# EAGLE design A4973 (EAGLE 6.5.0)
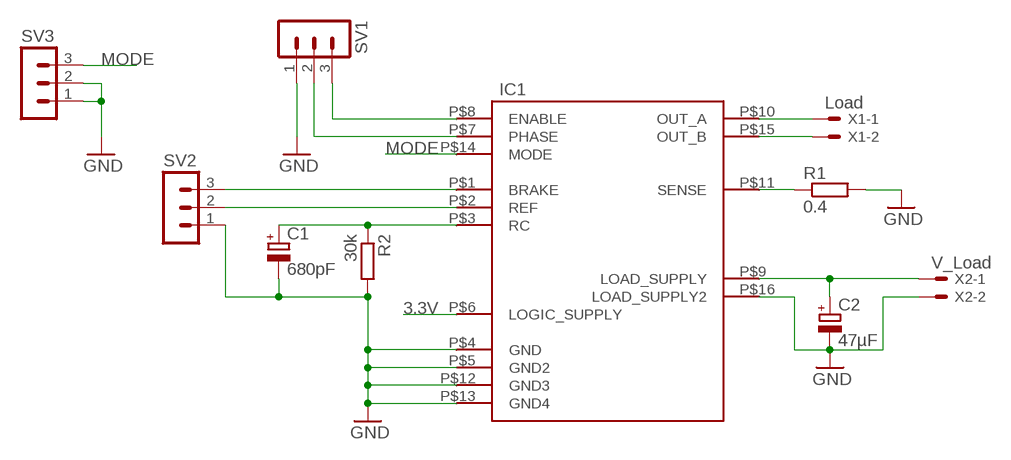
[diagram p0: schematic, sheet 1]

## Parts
C1  680pF  CPOL-EU153CLV-0405  [153CLV-0405]
C2  47µF  CPOL-EU153CLV-0405  [153CLV-0405]
IC1  A4973  [SOICW-16]
R1  0.4  R-EU_R1206  [R1206]
R2  30k  R-EU_R1206  [R1206]
SV1  MA03-1  [MA03-1]
SV2  MA03-1  [MA03-1]
SV3  MA03-1  [MA03-1]
X1  Load  22-23-2021  [22-23-2021]
X2  V_Load  22-23-2021  [22-23-2021]

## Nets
3.3V: IC1.P$6(LOGIC_SUPPLY)
GND: C1.- C2.- IC1.P$4(GND) IC1.P$5(GND2) IC1.P$12(GND3) IC1.P$13(GND4) IC1.P$16(LOAD_SUPPLY2) R1.2 R2.2 SV1.1 SV2.1 SV3.1 SV3.2 X2.2
MODE: IC1.P$14(MODE) SV3.3
N$1: IC1.P$8(ENABLE) SV1.3
N$2: IC1.P$7(PHASE) SV1.2
N$4: IC1.P$10(OUT_A) X1.1
N$5: IC1.P$15(OUT_B) X1.2
N$6: IC1.P$11(SENSE) R1.1
N$7: C1.+ IC1.P$3(RC) R2.1
N$8: C2.+ IC1.P$9(LOAD_SUPPLY) X2.1
N$9: IC1.P$1(BRAKE) SV2.3
N$10: IC1.P$2(REF) SV2.2

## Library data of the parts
C1 C2 = rcl:CPOL-EU: POLARIZED CAPACITOR, European symbol
IC1 = robust:A4973
R1 R2 = rcl:R-EU_: RESISTOR, European symbol
SV1-SV3 = con-lstb:MA03-1: PIN HEADER; OC_FARNELL: unknown; OC_NEWARK: unknown
X1 X2 = con-molex:22-23-2021: .100" (2.54mm) Center Header - 2 Pin; MF: MOLEX; MPN: 22-23-2021; OC_FARNELL: 1462926; OC_NEWARK: 25C3832

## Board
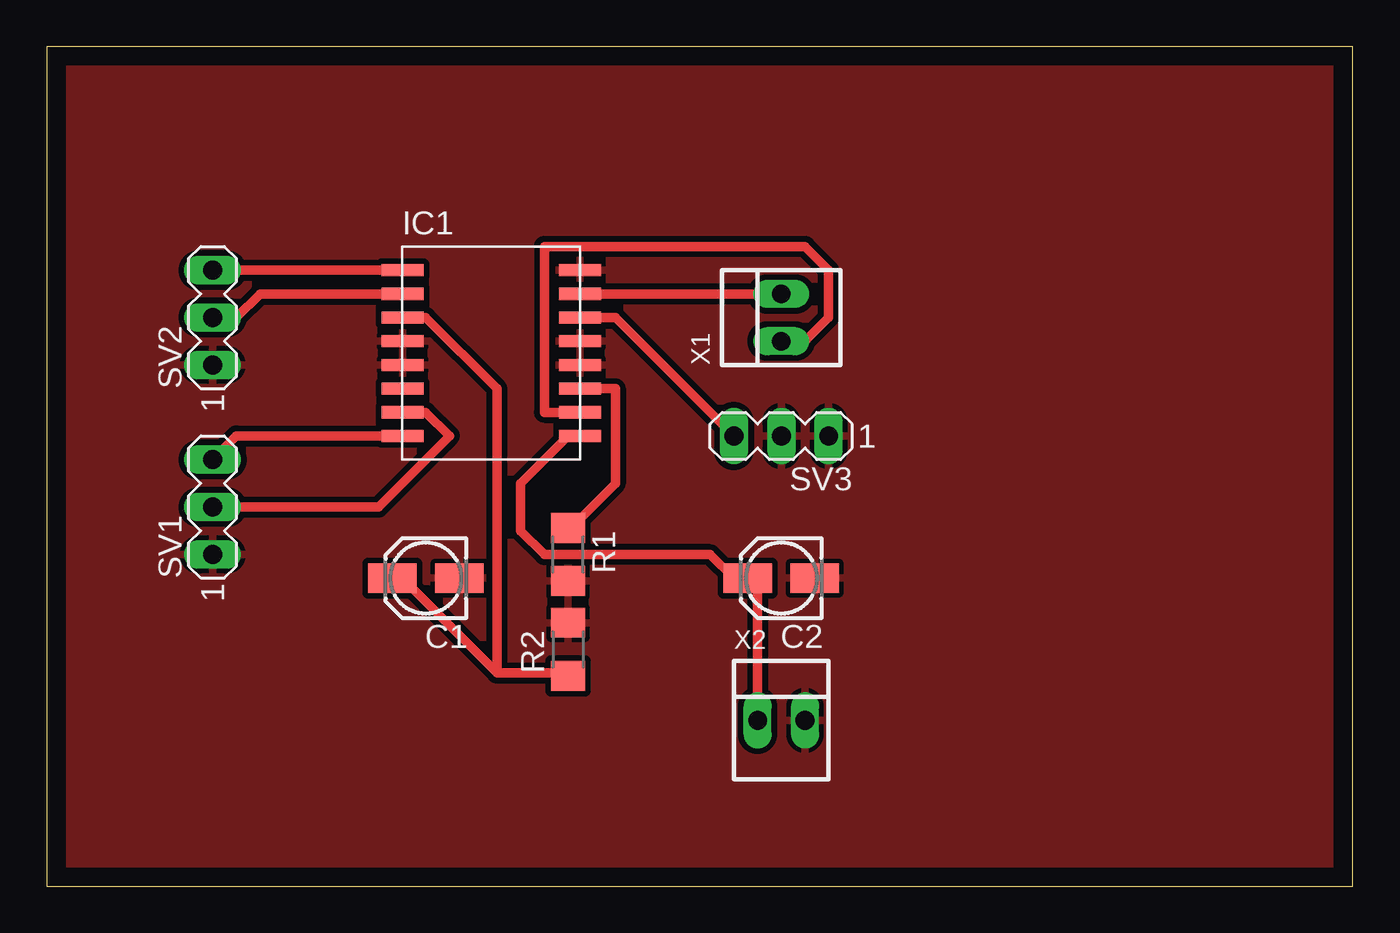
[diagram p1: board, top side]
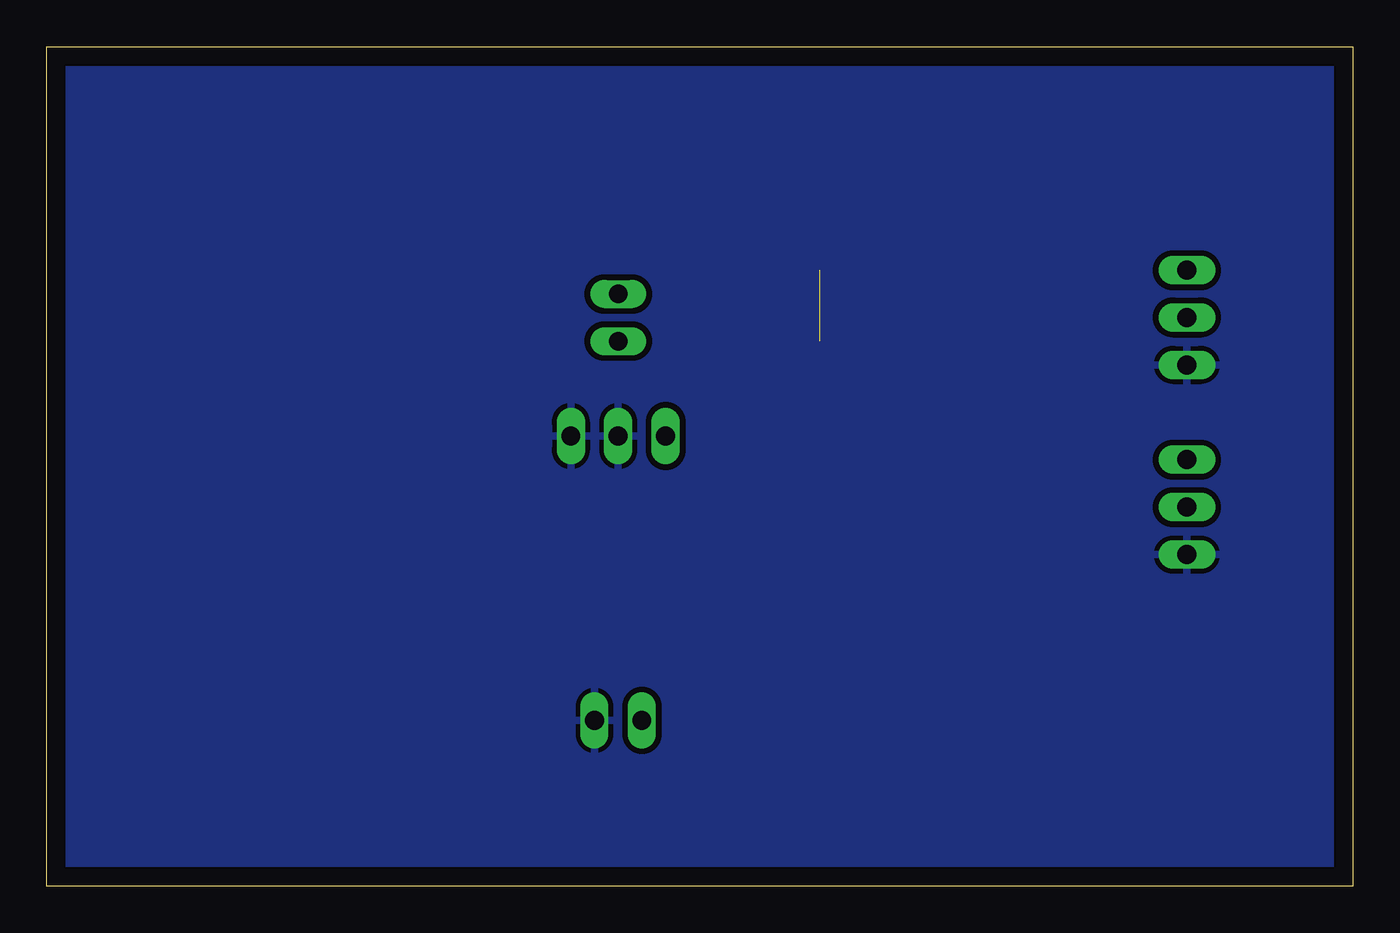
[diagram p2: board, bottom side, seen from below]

Size 70 x 45 mm. Coordinates in mm from the lower left corner, seen from the top.
Outline: 0,0 70,0 70,45 0,45 0,0
Copper layers (1*16): Top 0.035mm / dielectric 1.5mm / Bottom 0.035mm
Design rules "default *": minimum track width 20mil, minimum drill 24mil, track to track 12mil, track to pad 12mil, pad to pad 12mil, via to via 12mil, smd to smd 12mil, copper to edge 40mil, drill to drill 8mil, minimum pad ring 10mil, minimum via ring 8mil, stop-mask expansion 4mil, vias tented up to drill 0mil, thermal gap 10mil

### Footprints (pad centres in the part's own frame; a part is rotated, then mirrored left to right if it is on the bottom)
153CLV-0405 = smd 2.6 x 1.6: + 1.8,0; - -1.8,0
SOICW-16 = smd 2.25 x 0.65: P$1 0.025,10.16; P$2 0.025,8.89; P$3 0.025,7.62; P$4 0.025,6.35; P$5 0.025,5.08; P$6 0.025,3.81; P$7 0.025,2.54; P$8 0.025,1.27; P$9 9.525,1.27; P$10 9.525,2.54; P$11 9.525,3.81; P$12 9.525,5.08; P$13 9.525,6.35; P$14 9.525,7.62; P$15 9.525,8.89; P$16 9.525,10.16
R1206 = smd 1.6 x 1.803: 1 -1.422,0; 2 1.422,0
MA03-1 = drill 1.016 long: 1 -2.54,0; 2 0,0; 3 2.54,0
22-23-2021 = drill 1 long: 1 -1.27,0; 2 1.27,0

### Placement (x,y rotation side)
C1  20.32,16.51 180 top
C2  39.37,16.51 180 top
IC1  19.05,22.86 0 top
R1  27.94,17.78 270 top
R2  27.94,12.7 90 top
SV1  8.89,20.32 90 top
SV2  8.89,30.48 90 top
SV3  39.37,24.13 180 top
X1  39.37,30.48 90 top
X2  39.37,8.89 0 top

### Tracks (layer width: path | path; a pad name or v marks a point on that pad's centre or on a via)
GND  (1 unrouted)
  pour Top: 0,0 69.85,0 69.85,45.72 0,45.72
  pour Bottom: 0,45.72 0,0 69.85,0 69.85,45.72
MODE
  Top 0.508: IC1.P$14 30.48,30.48 SV3.3
N$1
  Top 0.508: IC1.P$8 10.16,24.13 SV1.3
N$2
  Top 0.508: SV1.2 17.78,20.32 21.59,24.13 20.32,25.4 IC1.P$7 19.05,25.4
N$4
  Top 0.508: IC1.P$10 26.67,25.4 26.67,34.29 40.64,34.29 41.91,33.02 41.91,30.48 40.64,29.21 X1.1
N$5
  Top 0.508: X1.2 IC1.P$15
N$6
  Top 0.508: IC1.P$11 30.48,26.67 30.48,21.59 27.94,19.05 R1.1
N$7
  Top 0.508: 24.13,11.43 27.94,11.43 R2.1 | 24.13,11.43 19.05,16.51 C1.+ | 24.13,11.43 24.13,26.67 20.32,30.48 IC1.P$3 19.05,30.48
N$8
  Top 0.508: IC1.P$9 27.94,24.13 25.4,21.59 25.4,19.05 26.67,17.78 35.56,17.78 36.83,16.51 C2.+ 38.1,16.51 X2.1
N$9
  Top 0.508: SV2.3 IC1.P$1
N$10
  Top 0.508: IC1.P$2 11.43,31.75 10.16,30.48 SV2.2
